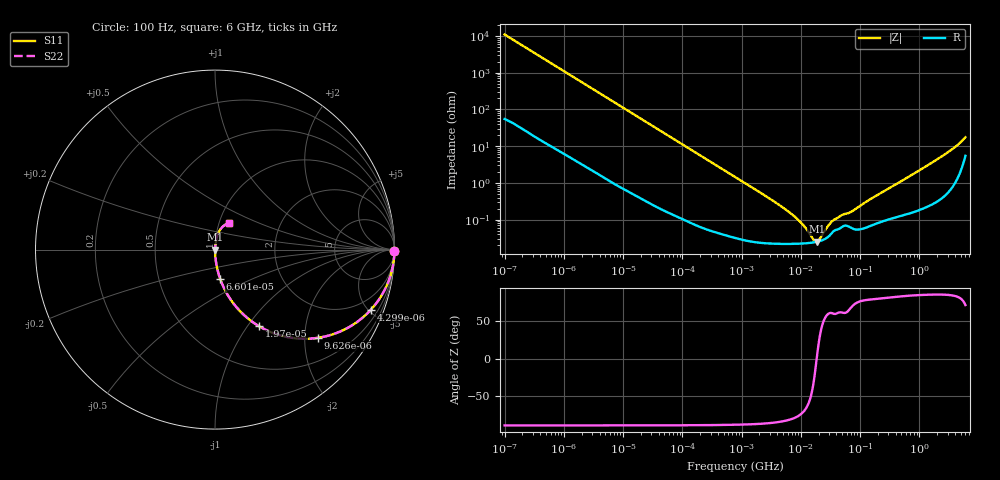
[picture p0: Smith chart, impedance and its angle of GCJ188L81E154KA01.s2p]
!Murata Part Number: GCJ188L81E154KA01
!These Parameters are Measured in Series Mode Connection
!Data Generated on Mar 13, 2026
!  o--ll--o
!Port1  Port2
!  o------o
!Operation Temp=25[degC], DC Bias Voltage=0[V]
!Freq. Start=100[Hz] Stop=6[GHz] 401[Steps]
# Hz S RI R 50
!Freq.(Hz) S11(Real) S11(Imag) S21(Real) S21(Imag) S12(Real) S12(Imag) S22(Real) S22(Imag)
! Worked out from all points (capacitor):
!   401 points, 100 Hz to 6 GHz, reference 50 ohm
!   read as one part in series: C = 144 nF near 109 Hz
!   lowest |Z| = 25.1 mohm at 18.61 MHz (marker M1)
!   series resonance near 18.55 MHz, so ESL is about 510 pH
!   S11 on the Smith chart (normalised r, x): 100 Hz: open; 4.299 kHz: 1.03, -5.19; 9.626 kHz: 1.01, -2.32; 19.7 kHz: 1.01, -1.14; 66 kHz: 1.00, -0.34; 6 GHz: 1.11, +0.34
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100  0.9999 -0.00909  0.000128 0.00909  0.000128 0.00909  0.9999 -0.00909
600  0.9968 -0.054  0.00322 0.054  0.00322 0.054  0.9968 -0.054
2008  0.9675 -0.1745  0.0325 0.1745  0.0325 0.1745  0.9675 -0.1745
4299  0.8692 -0.3343  0.1308 0.3343  0.1308 0.3343  0.8692 -0.3343
6433  0.7496 -0.4303  0.2504 0.4303  0.2504 0.4303  0.7496 -0.4303
9626  0.5741 -0.4914  0.4259 0.4914  0.4259 0.4914  0.5741 -0.4914
19704  0.2462 -0.4275  0.7538 0.4275  0.7538 0.4275  0.2462 -0.4275
40335  0.0738 -0.2578  0.9262 0.2578  0.9262 0.2578  0.0738 -0.2578
66005  0.0296 -0.1655  0.9704 0.1655  0.9704 0.1655  0.0296 -0.1655
184852  0.0044 -0.061  0.9956 0.061  0.9956 0.061  0.0044 -0.061
774597  0.000536 -0.0147  0.9995 0.0147  0.9995 0.0147  0.000536 -0.0147
6644369  0.000222 -0.00151  0.9998 0.00151  0.9998 0.00151  0.000222 -0.00151
1.087309e7  0.000226 -0.000696  0.9998 0.000696  0.9998 0.000696  0.000226 -0.000696
1.555665e7  0.000238 -0.000221  0.9998 0.000221  0.9998 0.000221  0.000238 -0.000221
1.86079e7  0.000251 3.9e-06  0.9997 -3.9e-06  0.9997 -3.9e-06  0.000251 3.9e-06
2.128304e7  0.000265 0.000174  0.9997 -0.000174  0.9997 -0.000174  0.000265 0.000174
3.045065e7  0.000368 0.000662  0.9996 -0.000662  0.9996 -0.000662  0.000368 0.000662
3.64232e7  0.0005 0.000864  0.9995 -0.000864  0.9995 -0.000864  0.0005 0.000864
7.129496e7  0.000596 0.00154  0.9994 -0.00154  0.9994 -0.00154  0.000596 0.00154
3.124326e8  0.00108 0.00717  0.9989 -0.00717  0.9989 -0.00717  0.00108 0.00717
2.34314e9  0.00632 0.0511  0.9937 -0.0511  0.9937 -0.0511  0.00632 0.0511
6e9  0.0754 0.1469  0.9246 -0.1469  0.9246 -0.1469  0.0754 0.1469
